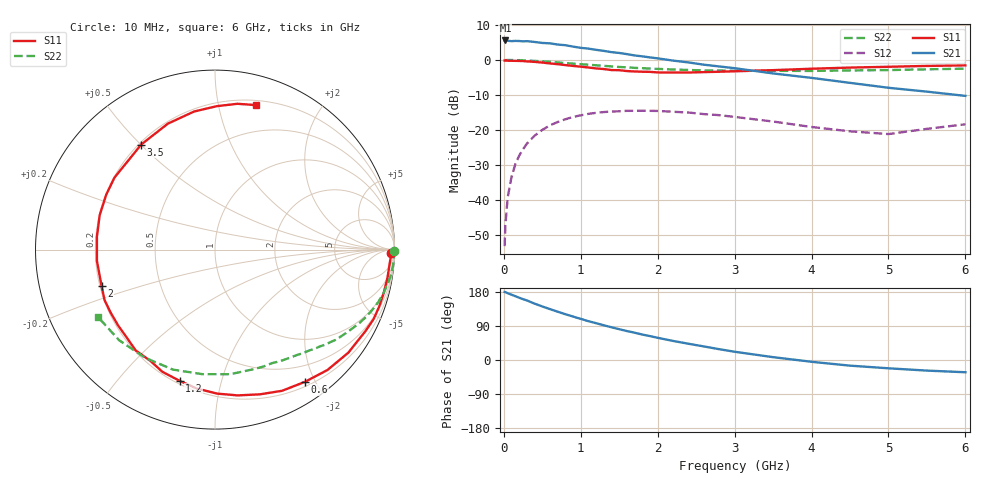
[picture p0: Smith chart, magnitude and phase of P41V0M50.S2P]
! SIEMENS Small Signal Semiconductors
! BFP182
! Si NPN RF Bipolar Junction Transistor in SOT143
! VCE = 1 V  IC = 0.5 mA
! Common Emitter S-Parameters:  March  1996
# GHz  S  MA  R  50
!  f  S11  S21  S12  S22
! GHz  MAG  ANG  MAG  ANG  MAG  ANG  MAG  ANG
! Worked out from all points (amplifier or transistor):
!   36 points, 10 MHz to 6 GHz, reference 50 ohm
!   highest |S21| = 5.6 dB at 20 MHz (marker M1)
!   |S21| within 3 dB of that: start of sweep to 1.306 GHz
!   unconditionally stable (mu >= 1): 2.881 GHz to end of sweep
!   at 250 MHz: K = 0.10, MSG = 15.4 dB, |S12| = -25.5 dB
!   at 1.4 GHz: K = 0.53, MSG = 8.5 dB, |S12| = -14.7 dB
!   at 6 GHz: K = 1.38, MAG = 0.4 dB, |S12| = -18.4 dB
!   S11 on the Smith chart (normalised r, x): 10 MHz: 52, -51; 600 MHz: 0.26, -1.86; 1.2 GHz: 0.22, -0.74; 2 GHz: 0.21, -0.15; 3.5 GHz: 0.21, +0.50; 6 GHz: 0.24, +1.29
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0.01  0.9805 -1.1  1.866 179.6  0.0022 87.1  0.9994 -0.3
0.02  0.9812 -1.9  1.898 179.2  0.0044 86.0  0.9928 -0.7
0.05  0.976 -4.8  1.879 176.2  0.0109 88.1  0.999 -1.8
0.1  0.9737 -9.4  1.855 172.3  0.0215 82.5  0.9968 -3.7
0.15  0.9706 -14.3  1.871 168.4  0.0326 80.4  0.995 -5.6
0.3  0.9533 -28.5  1.854 157.1  0.0641 71.2  0.9815 -11.0
0.4  0.939 -37.7  1.806 148.7  0.0831 65.1  0.97 -14.4
0.6  0.8913 -55.7  1.726 134.3  0.1166 53.5  0.939 -20.9
0.8  0.8442 -72.8  1.624 120.8  0.1423 43.0  0.9034 -26.8
1.1  0.7803 -97.6  1.451 102.4  0.1701 29.2  0.854 -34.3
1.2  0.7571 -105.1  1.394 97.1  0.1761 24.6  0.8392 -36.8
1.4  0.717 -120.1  1.293 86.3  0.1835 17.1  0.809 -41.0
1.6  0.694 -135.2  1.211 76.4  0.1879 10.5  0.7846 -44.7
2  0.6635 -162.3  1.054 58.6  0.1872 -0.6  0.7454 -51.8
2.2  0.6609 -174.5  0.979 50.3  0.1822 -5.8  0.731 -55.8
2.8  0.6789 153.2  0.808 28.5  0.163 -17.7  0.7053 -67.3
3.5  0.7153 125.1  0.642 7.5  0.1322 -25.0  0.6994 -83.1
4  0.7494 110.5  0.555 -4.7  0.1105 -23.8  0.6976 -95.8
4.5  0.7782 98.6  0.471 -14.9  0.0958 -18.4  0.7084 -109.3
5  0.7991 89.3  0.401 -21.9  0.0875 -4.5  0.7175 -122.9
5.5  0.8218 81.3  0.353 -28.0  0.1039 4.6  0.7351 -136.6
6  0.8365 74.3  0.307 -32.3  0.1208 7.6  0.7517 -149.8
